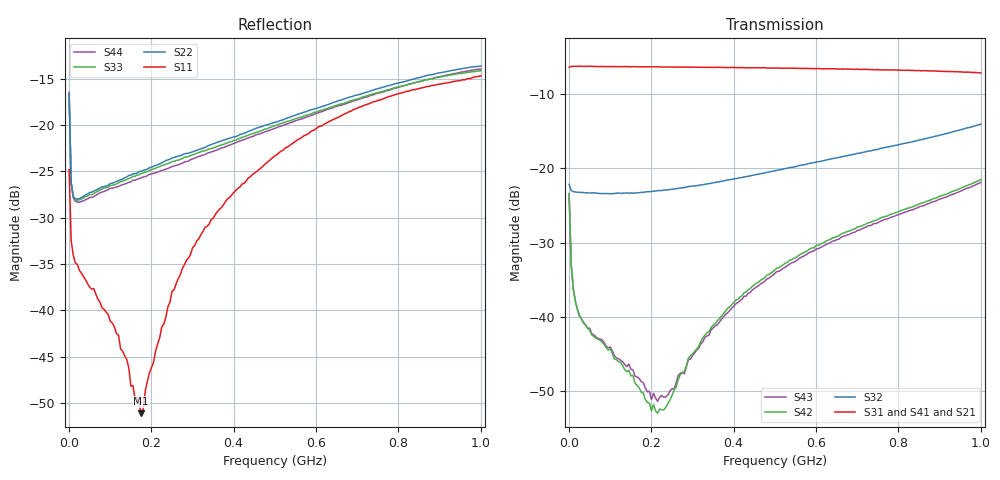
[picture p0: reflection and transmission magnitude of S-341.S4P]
!Agilent Technologies,E5071B,MY42300999,A.09.10
!Date: Thu Apr 13 17:04:38 2023
!Data & Calibration Information:
!Freq	S11:SOLT4(ON)	S12:SOLT4(ON)	S13:SOLT4(ON)	S14:SOLT4(ON)
!	S21:SOLT4(ON)	S22:SOLT4(ON)	S23:SOLT4(ON)	S24:SOLT4(ON)
!	S31:SOLT4(ON)	S32:SOLT4(ON)	S33:SOLT4(ON)	S34:SOLT4(ON)
!	S41:SOLT4(ON)	S42:SOLT4(ON)	S43:SOLT4(ON)	S44:SOLT4(ON)
# Hz S RI R 50
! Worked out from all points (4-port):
!   201 points, 1 MHz to 1 GHz, reference 50 ohm
!   strongest paths, dB at 1 MHz, 250.8 MHz, 500.5 MHz, 750.2 MHz, 1 GHz:
!     S31: -6.4, -6.3, -6.5, -6.7, -7.1
!     S41: -6.4, -6.4, -6.5, -6.7, -7.1
!     S21: -6.4, -6.4, -6.5, -6.8, -7.2
!     S32: -22.1, -22.8, -20.3, -17.4, -14.0
!     S42: -23.4, -50.5, -33.6, -26.8, -21.5
!     S43: -23.4, -49.7, -34.1, -27.3, -21.9
!   lowest |S11| = -51.1 dB at 175.8 MHz (marker M1), VSWR 1.01, Z = 50.2 + j0.224 ohm
!   |S11| at or under -10 dB: start of sweep to end of sweep
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1000000  -0.0372 0.0438  0.4785 0.0195  0.4788 0.019  0.4776 0.0196
         0.4784 0.0201  -0.0619 0.1339  -0.0782 0.00013  0.051 -0.0448
         0.479 0.0205  -0.0781 4.82e-05  -0.0619 0.134  0.051 -0.0449
         0.4777 0.0205  0.0507 -0.0446  0.0509 -0.0448  -0.0639 0.136
5995000  -0.0199 0.0129  0.4868 -0.00447  0.486 -0.00315  0.4862 -0.00447
         0.4873 -0.00455  0.0203 0.0447  -0.071 0.004  0.0143 -0.0178
         0.486 -0.00421  -0.0711 0.00404  0.0203 0.0444  0.0143 -0.0177
         0.4862 -0.00456  0.0143 -0.0178  0.0143 -0.0176  0.0189 0.0451
2.5975e7  -0.0145 0.00764  0.4857 -0.0379  0.485 -0.0392  0.4846 -0.0379
          0.4864 -0.0388  0.0362 0.0173  -0.0686 0.00788  0.00767 -0.00655
          0.4866 -0.0381  -0.0688 0.00794  0.036 0.0162  0.00758 -0.00667
          0.4853 -0.0394  0.00764 -0.00664  0.00773 -0.00671  0.0349 0.0159
1.75825e8  0.00167 0.00223  0.413 -0.2492  0.4158 -0.2465  0.4135 -0.2473
           0.4141 -0.2503  0.0563 -0.00279  -0.0588 0.0362  0.000191 -0.0032
           0.4161 -0.2467  -0.0589 0.0361  0.0538 -0.00953  0.000208 -0.00361
           0.4135 -0.2477  0.000216 -0.00313  0.000227 -0.00368  0.051 -0.00995
2.5075e8  0.0108 -0.00673  0.3435 -0.3354  0.3485 -0.3312  0.3454 -0.3333
          0.3437 -0.3358  0.0647 -0.0148  -0.0534 0.0491  -0.00291 -0.000133
          0.3483 -0.3328  -0.0531 0.0493  0.0593 -0.0225  -0.00322 -0.000804
          0.345 -0.3323  -0.00297 -5.81e-05  -0.00318 -0.000844  0.0553 -0.0225
4.2058e8  0.014 -0.0459  0.1219 -0.4582  0.1313 -0.4572  0.128 -0.4581
          0.1218 -0.4583  0.072 -0.053  -0.0355 0.0792  -0.0055 0.0128
          0.1307 -0.4586  -0.0357 0.0793  0.061 -0.06  -0.00616 0.0116
          0.1269 -0.4568  -0.0054 0.0128  -0.00624 0.0116  0.0567 -0.0605
1e9  -0.0975 0.1566  -0.4034 0.1658  -0.4166 0.1435  -0.4168 0.1475
     -0.4041 0.1663  -0.1093 -0.1765  0.128 0.1523  0.0724 0.0424
     -0.4156 0.1434  0.1282 0.1519  -0.0943 -0.1716  0.0682 0.0426
     -0.418 0.1484  0.0726 0.0426  0.0683 0.0428  -0.1134 -0.165
